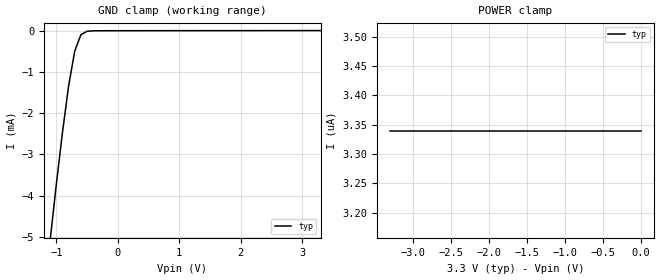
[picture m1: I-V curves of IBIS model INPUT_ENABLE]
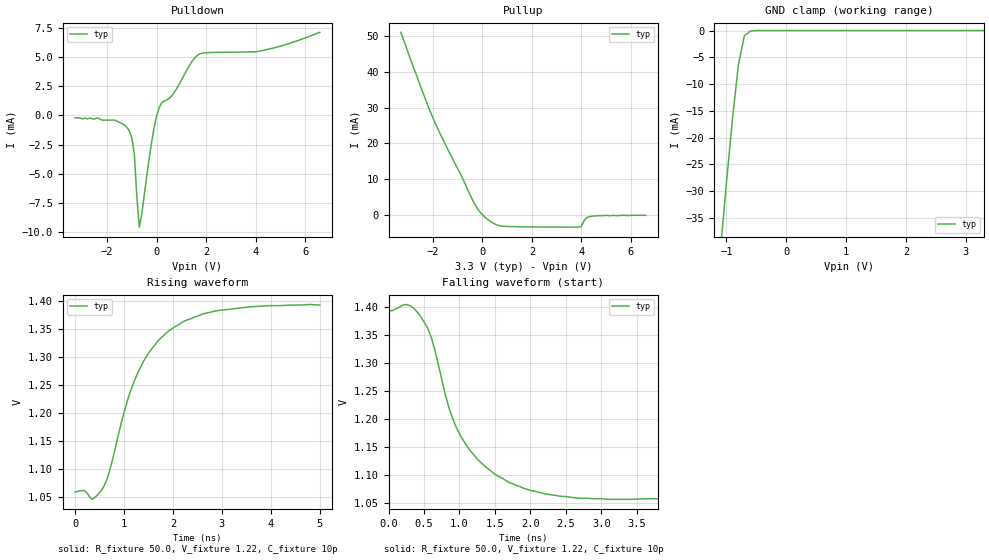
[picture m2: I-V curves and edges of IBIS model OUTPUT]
|   Texas Instruments Incorporated
|   Data Transmissions Products
|   IBIS Model for SN65LVDS391
|   16D SOIC Package
[IBIS Ver]   3.2
[Comment char]   |_char
[File name]   lvds391.ibs
[File Rev]   1.0
[Date]   11Oct00
[Source]   File originated at Texas Instruments Incorporated.
   Data Transmission Products Group.
[Notes]   Model revved in Nov02 to fix common-mode bug  -TMF-
[Disclaimer]
(C) Copyright Texas Instruments Incorporated 2000
   All rights reserved
  Texas Instruments Incorporated hereby grants the user of this IBIS
model a non-exclusive, nontransferable license to use this IBIS model
under the following terms.  Before using this IBIS model, the user
should read this license.  If the user does not accept these terms,
the IBIS model should be returned to Texas Instruments within 30 days.
  The user is granted this license only to use the IBIS model and
is not granted rights to sell, load, rent, lease or license the IBIS
model in whole or in part, or in modified form to anyone other than
user.  User may modify the IBIS model to suit its specific applications
but rights to derivative works and such modifications shall belong to
Texas Instruments.
  This IBIS model is provided on an "AS IS" basis and Texas Instruments
makes absolutely no warranty with respect to the information contained
herein.  TEXAS INSTRUMENTS DISCLAIMS AND CUSTOMER WAIVES ALL WARRANTIES,
EXPRESS OR IMPLIED, INCLUDING WARRANTIES OF MERCHANTABILITY OR FITNESS
FOR A PARTICULAR PURPOSE. The entire risk as to quality and performance
is with the Customer. ACCORDINGLY, IN NO EVENT SHALL THE COMPANY BE LIABLE
FOR ANY DAMAGES, WHETHER IN CONTRACT OR TORT,INCLUDING ANY LOST PROFITS
OR OTHER INCIDENTAL, CONSEQUENTIAL, EXEMPLARY, OR PUNITIVE DAMAGES ARISING
OUT OF THE USE OR APPLICATION OF THE IBIS model provided in this package.
Further, Texas Instruments reserves the right to discontinue or make changes
without notice to any product herein to improve reliability, function, or
design. Texas Instruments does not convey any license under patent rights
or any other intellectual property rights, including those of third parties.
Contact Texas Instruments at ATTN:DATA TRANSMISSIONS
[Copyright]   Copyright 2000, Texas Instruments, All Rights Reserved
[Component]   LVDS391D
[Manufacturer]  Texas Instruments Incorporated
[Package]
|   typ   min   max
R_pkg   0.035   0.030   0.040
L_pkg   2.181nH   1.231nH   3.257nH
C_pkg   0.322pF   0.163pF   0.546pF
[Pin]   signal_name   model_name   R_pin   L_pin   C_pin
1   EN1,2   INPUT_ENABLE   0.040   3.251n   0.546p
2   1A   INPUT_ENABLE   0.039   2.561n   0.393p
3   2A   INPUT_ENABLE   0.030   1.681n   0.186p
4   VCC   POWER   0.030   1.231n   0.163p
5   GND   GND   0.030   1.231n   0.163p
6   3A   INPUT_ENABLE   0.030   1.681n   0.186p
7   4A   INPUT_ENABLE   0.039   2.564n   0.393p
8   EN3,4   INPUT_ENABLE   0.040   3.257n   0.545p
9   4Z   OUTPUT   0.040   3.247n   0.546p
10   4Y   OUTPUT   0.039   2.558n   0.394p
11   3Z   OUTPUT   0.030   1.681n   0.187p
12   3Y   OUTPUT   0.030   1.231n   0.163p
13   2Z   OUTPUT   0.030   1.231n   0.163p
14   2Y   OUTPUT   0.030   1.681n   0.187p
15   1Z   OUTPUT   0.039   2.558n   0.394p
16   1Y   OUTPUT   0.040   3.246n   0.546p
[Diff_pin]   inv_pin   vdiff   tdelay_typ   tdelay_min   tdelay_max
| The 'xY' pin is Diff_pin and the 'xZ' pin is the inv_pin
16   15   NA   0 0 0
14   13   NA   0 0 0
12   11   NA   0 0 0
10   9   NA   0 0 0
| Models and submodels in the file (2): INPUT_ENABLE (Input), OUTPUT (3-state)
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|   Driver Input / Enable Model
[Model]   INPUT_ENABLE
Model_type   Input
|Signals   EN1,2 EN3,4, 1A,2A,3A,4A
Vinh = 2.0
Vinl = 0.8
|   typ   min   max
C_comp   1.0pF   NA   NA
|   typ   min   max
[Temperature Range]   25.0   NA   NA
[Voltage range]   3.3V   3.0V   3.6V
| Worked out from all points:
|   GND clamp passes 1 mA (typ) near -0.76 V on its own axis
[GND_clamp]
|   Voltage   I(typ)   I(min)   I(max)
-3.3V     -43.1mA    NA         NA
-1.1V     -5.08mA    NA         NA
-1V       -3.73mA    NA         NA
-900mV    -2.47mA    NA         NA
-800mV    -1.34mA    NA         NA
-700mV    -493uA     NA         NA
-600mV    -98.5uA    NA         NA
-500mV    -13.3uA    NA         NA
3.3V      3.34uA     NA         NA
[Power_clamp]
| Note that the[POWER_clamp]voltage table is referenced to Vcc
| and is calculated using Vtable=Vcc - Vmeasured.
|   Voltage   I(typ)   I(min)   I(max)
-3.3V     3.34uA     NA         NA
-2.7V     3.34uA     NA         NA
-2V       3.34uA     NA         NA
-800mV    3.34uA     NA         NA
0V        3.34uA     NA         NA
|   Driver Output Model
[Model]   OUTPUT
Model_type   3-state
| Signals   1Y,1Z,2Y,2Z,3Y,3Z,4Y,4Z
Vmeas = 1.2V   |Reference voltage for timing measurements
Cref = 10pF   |Timing specification test load capacitance value
Rref = 50   |Note: 50 Ohm load; single ended configuration
Vref = 1.20V   |Timing specification test load voltage
| variable   typ   min   max
C_comp   1.0pF   NA   NA
|   typ   min   max
[Temperature Range]   25.0   NA   NA
[Voltage range]   3.3V   3.0V   3.6V
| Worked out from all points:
|   slope of the pulldown table from 0 to 0.495 V, typ, clamps not added: 335 ohm
|   slope of the pullup table from 0 to 0.495 V, typ, clamps not added: 192 ohm
|   GND clamp passes 1 mA (typ) near -0.70 V on its own axis
|   rising waveform, R_fixture 50.0, V_fixture 1.22, C_fixture 10p: 20-80 % time 879ps typ, NA min, NA max; typ from 1.06 V to 1.39 V
|   falling waveform, R_fixture 50.0, V_fixture 1.22, C_fixture 10p: 20-80 % time 611ps typ, NA min, NA max; typ from 1.39 V to 1.06 V
[Pulldown]
|   Voltage   I(typ)   I(min)   I(max)
-3.3V     -200uA     NA         NA
-1.7V     -400uA     NA         NA
-1.1V     -1.34mA    NA         NA
-900mV    -3.37mA    NA         NA
-800mV    -6.98mA    NA         NA
-700mV    -9.59mA    NA         NA
-200mV    -2.26mA    NA         NA
100mV     664uA      NA         NA
700mV     1.94mA     NA         NA
1.6V      5.08mA     NA         NA
4.3V      5.58mA     NA         NA
6.6V      7.14mA     NA         NA
[Pullup]
|   Voltage   I(typ)   I(min)   I(max)
| Note that the[Pullup]voltage table is referenced to Vcc
| and is calculated using Vtable=Vcc - Vmeasured.
-3.3V     51mA       NA         NA
-2.2V     30.4mA     NA         NA
-1.7V     22.5mA     NA         NA
-300mV    2.87mA     NA         NA
-100mV    817uA      NA         NA
300mV     -1.72mA    NA         NA
900mV     -3.18mA    NA         NA
3.9V      -3.41mA    NA         NA
4V        -3.21mA    NA         NA
4.2V      -820uA     NA         NA
4.4V      -370uA     NA         NA
6.6V      -100uA     NA         NA
[GND_clamp]
|   Voltage   I(typ)   I(min)   I(max)
| Outputs in High Impedance (off)
-3.3V     -347mA     NA         NA
-1.1V     -41.1mA    NA         NA
-1V       -28.5mA    NA         NA
-900mV    -16.6mA    NA         NA
-800mV    -6.42mA    NA         NA
-700mV    -997uA     NA         NA
-600mV    -101uA     NA         NA
3.3V      -64pA      NA         NA
[POWER_clamp]
|   Voltage   I(typ)   I(min)   I(max)
| Note that the [POWER_clamp] voltage table is referenced to Vcc
| and is calculated using Vtable = Vcc - Vmeasured.
| Outputs in Tri-state.
-3.3V     0A         NA         NA
0V        0A         NA         NA
[Ramp]
|   typ   min   max
dV/dt_r   0.202/870ps   NA   NA
dV/dt_f   0.199/749ps   NA   NA
R_load = 50ohm
[Rising Waveform]
R_fixture = 50.0
V_fixture = 1.22
C_fixture = 10p
L_fixture = 0n
|   V(typ)   V(min)   V(max)
0s        1.059V     NA         NA
350ps     1.046V     NA         NA
550ps     1.063V     NA         NA
700ps     1.095V     NA         NA
1.05ns    1.216V     NA         NA
1.25ns    1.265V     NA         NA
1.5ns     1.306V     NA         NA
1.9ns     1.345V     NA         NA
2.9ns     1.382V     NA         NA
5ns       1.392V     NA         NA
[Falling Waveform]
R_fixture = 50.0
V_fixture = 1.22
C_fixture = 10p
L_fixture = 0n
|   V(typ)   V(min)   V(max)
0s        1.393V     NA         NA
250ps     1.404V     NA         NA
450ps     1.383V     NA         NA
600ps     1.346V     NA         NA
850ps     1.22V      NA         NA
1ns       1.173V     NA         NA
1.25ns    1.128V     NA         NA
1.7ns     1.086V     NA         NA
2.7ns     1.058V     NA         NA
5ns       1.061V     NA         NA
